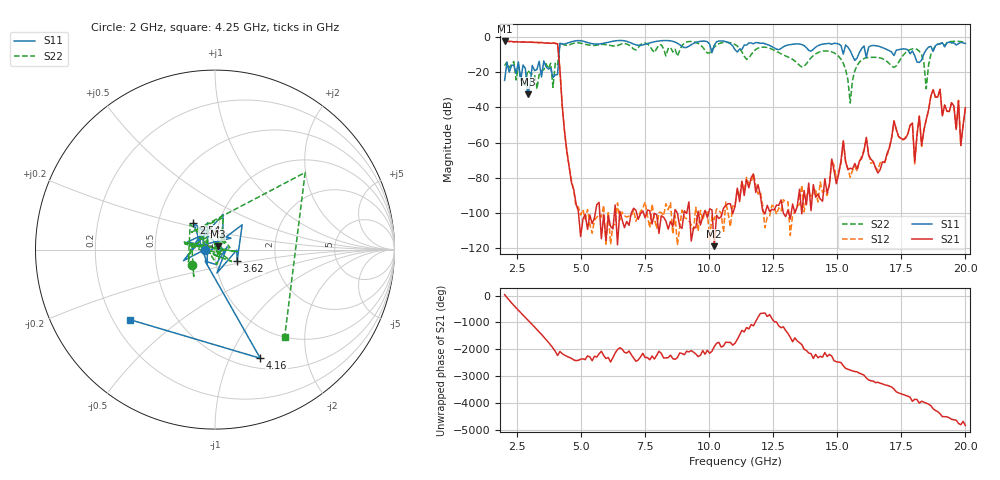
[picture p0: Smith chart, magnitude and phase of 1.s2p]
!Keysight Technologies,N5234A,MY52241180,A.10.60.03
!Date: Friday, January 20, 2023 09:32:41
!Correction: S11(Full 2 Port(1,2))
!S21(Full 2 Port(1,2))
!S12(Full 2 Port(1,2))
!S22(Full 2 Port(1,2))
!S2P File: Measurements: S11, S21, S12, S22:
# Hz S  dB  R 50
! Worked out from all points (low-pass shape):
!   201 points, 2 GHz to 20 GHz, reference 50 ohm
!   highest |S21| = -2.61 dB at 2 GHz (marker M1); lowest = -118.7 dB at 10.19 GHz (marker M2)
!   |S21| within 3 dB of the highest: start of sweep to 4.08 GHz
!   lowest |S11| = -32.6 dB at 2.9 GHz (marker M3), VSWR 1.05, Z = 51.4 + j1.92 ohm
!   |S11| at or under -10 dB: start of sweep to 4.128 GHz; 15.56 GHz to 15.83 GHz (265.6 MHz wide, 1.69 % of centre); 17.99 GHz to 18.37 GHz (376.7 MHz wide, 2.07 % of centre)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
!   |S22| runs from -37.6 to -2.6 dB; largest |S21 - S12| = 0.0003
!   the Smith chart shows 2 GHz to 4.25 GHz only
!   S11 on the Smith chart (normalised r, x): 2 GHz: 0.89, -0.00; 2.54 GHz: 0.75, +0.23; 3.62 GHz: 1.27, -0.17; 4.16 GHz: 0.62, -1.31; 4.25 GHz: 0.27, -0.34
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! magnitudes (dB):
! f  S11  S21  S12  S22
! 2 GHz  -24.8  -2.6  -2.6  -16.4
! 2.54 GHz  -14.3  -3.0  -3.0  -16.7
! 2.9 GHz  -32.6  -3.1  -3.1  -19.1
! 3.62 GHz  -17.1  -3.7  -3.7  -15.3
! 4.16 GHz  -3.7  -18.6  -18.6  -3.6
! 4.25 GHz  -4.2  -39.1  -39.1  -4.1
! 4.61 GHz  -2.9  -82.5  -81.4  -4.2
! 5.06 GHz  -2.5  -103.3  -98.0  -4.0
! 8.03 GHz  -2.4  -111.5  -99.5  -4.7
! 10.19 GHz  -4.9  -118.7  -103.6  -5.9
! 11 GHz  -7.4  -96.1  -96.0  -4.4
! 14.06 GHz  -7.2  -83.8  -88.3  -10.7
! 15.23 GHz  -9.9  -59.0  -59.0  -15.1
! 15.5 GHz  -7.9  -74.5  -79.7  -37.6
! 17.03 GHz  -7.9  -63.2  -62.5  -15.3
! 17.93 GHz  -8.1  -49.0  -49.0  -6.9
! 18.02 GHz  -10.7  -71.0  -72.0  -6.9
! 18.47 GHz  -7.4  -47.0  -47.1  -29.5
! 19.01 GHz  -4.0  -29.9  -29.8  -4.0
! 19.73 GHz  -3.9  -36.2  -36.2  -2.7
! 19.82 GHz  -3.2  -61.6  -61.7  -2.8
! 20 GHz  -3.8  -40.3  -40.3  -3.4
